(* Logix 5000 AddOnInstructionDefinition export B256_CtoS; software revision 30.00 *)

ADD_ON_INSTRUCTION D_SHR   (* revision 1.0, vendor Ken Fischer, NSWCPD, C512 *)
// DINT bit shift right of the 32-bit argument Inp_A by Inp_B bits with paddding by zeros on the right
// Revision note:
// Rev1.0: TBD - Initial Release
VAR_IN_OUT
   Inp_A : DINT; {required}   // 64-bit Integer to be right circular rotated
END_VAR
VAR_INPUT
   Inp_B : INT; {required}   // Number of bits to shift
END_VAR
VAR_IN_OUT
   Out : DINT; {required}   // Result
END_VAR
VAR
   BSR_Cntrl : CONTROL := (LEN := 32);
   ONS : BOOL;
   Source_Bit : BOOL;
   Wrk_InpA : DINT[2];
END_VAR

ROUTINE Logic   (* ladder *)
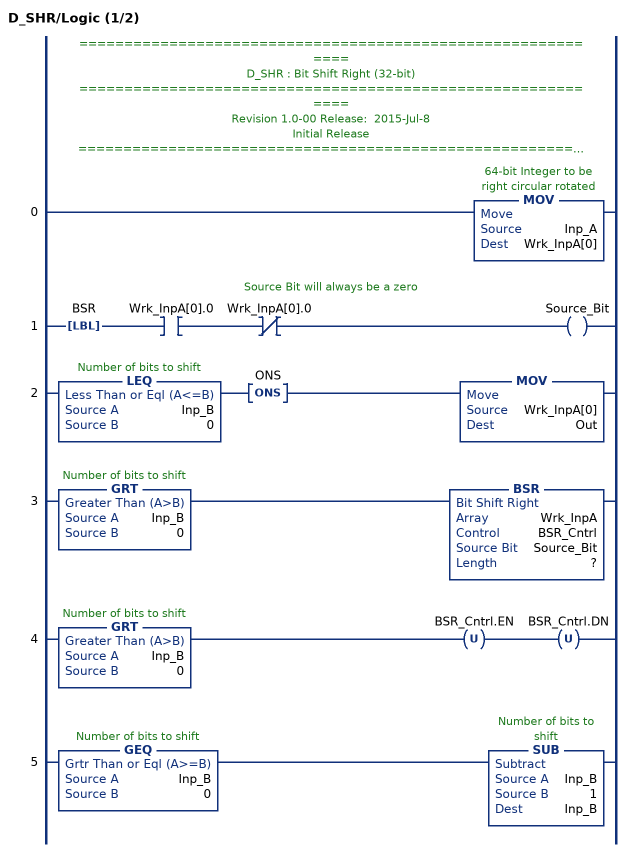
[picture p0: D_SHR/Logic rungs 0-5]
   // ============================================================
   // D_SHR : Bit Shift Right (32-bit)
   // ============================================================
   // Revision 1.0-00 Release:  2015-Jul-8
   // Initial Release
   // ============================================================
   // Performs a right bit shift of the 32-bit argument Inp_A by the
   // number of bits defined in the 16-bit argument Inp_B, with padding by zeros.
   0: MOV(Inp_A,Wrk_InpA[0]);
   // Source Bit will always be a zero
   1: LBL(BSR)XIC(Wrk_InpA[0].0)XIO(Wrk_InpA[0].0)OTE(Source_Bit);
   2: LEQ(Inp_B,0)ONS(ONS)MOV(Wrk_InpA[0],Out);
   3: GRT(Inp_B,0)BSR(Wrk_InpA,BSR_Cntrl,Source_Bit,?);
   4: GRT(Inp_B,0)OTU(BSR_Cntrl.EN)OTU(BSR_Cntrl.DN);
   5: GEQ(Inp_B,0)SUB(Inp_B,1,Inp_B);
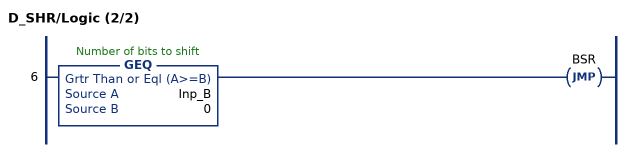
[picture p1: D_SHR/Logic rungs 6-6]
   6: GEQ(Inp_B,0)JMP(BSR);
END_ROUTINE
END_ADD_ON_INSTRUCTION

ADD_ON_INSTRUCTION B256_CtoS   (* revision 1.0 20170916, vendor Kenneth A. Fischer *)
// Convert 256-bit value using 22 12-bit pieces into 64 hex big endian string characters
// Revision note:
// Rev1.0: 20170916 - Initial Release
VAR_IN_OUT
   Inp_C : DINT[22]; {required}
   Out_S : STRING; {required}
END_VAR
VAR
   byte : DINT[3];
   i : INT;
   j : INT;
   k : DINT;
   D_SHR : D_SHR;
END_VAR

ROUTINE Logic   (* ladder *)
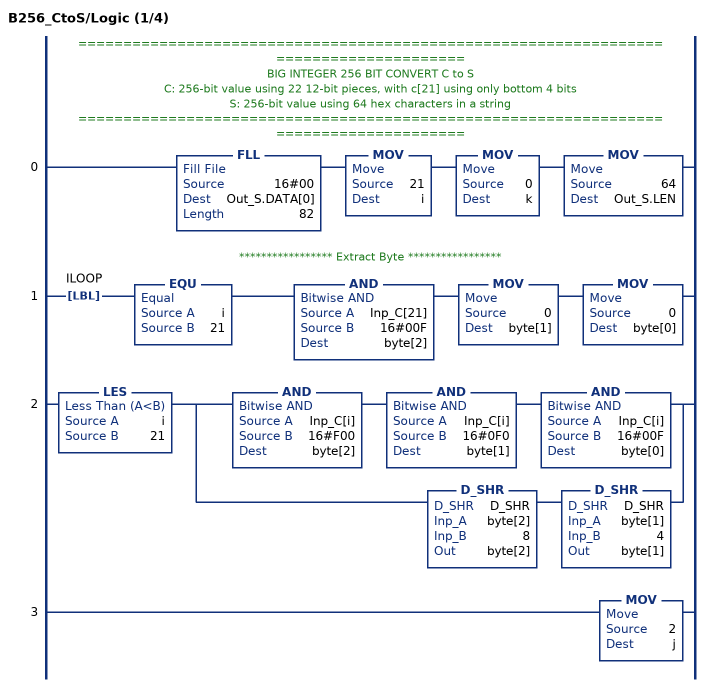
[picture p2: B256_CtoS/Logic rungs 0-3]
   // ======================================================================================
   // BIG INTEGER 256 BIT CONVERT C to S
   // C: 256-bit value using 22 12-bit pieces, with c[21] using only bottom 4 bits
   // S: 256-bit value using 64 hex characters in a string
   // ======================================================================================
   0: FLL(16#00,Out_S.DATA[0],82)MOV(21,i)MOV(0,k)MOV(64,Out_S.LEN);
   // ***************** Extract Byte *****************
   1: LBL(ILOOP)EQU(i,21)AND(Inp_C[21],16#00F,byte[2])MOV(0,byte[1])MOV(0,byte[0]);
   2: LES(i,21)[AND(Inp_C[i],16#F00,byte[2]) AND(Inp_C[i],16#0F0,byte[1]) AND(Inp_C[i],16#00F,byte[0]) ,D_SHR(D_SHR,byte[2],8,byte[2]) D_SHR(D_SHR,byte[1],4,byte[1]) ];
   3: MOV(2,j);
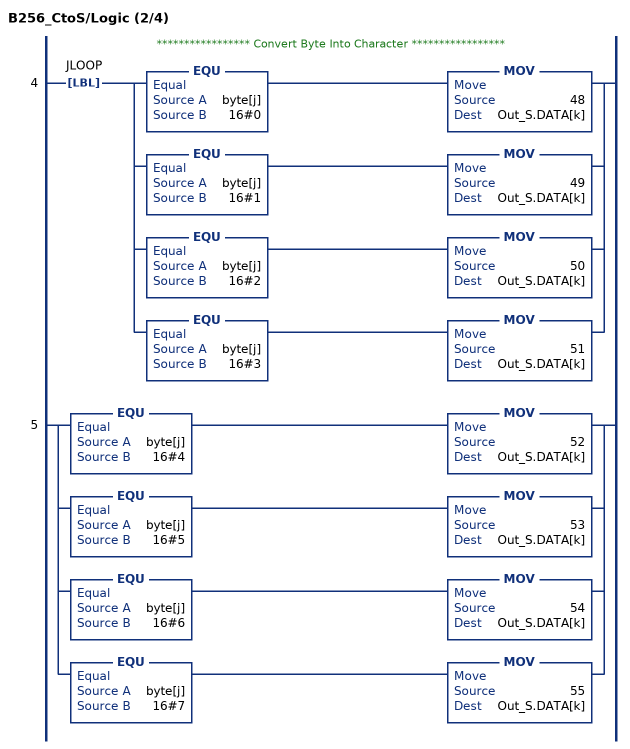
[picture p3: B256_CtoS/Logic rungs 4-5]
   // ***************** Convert Byte Into Character *****************
   4: LBL(JLOOP)[EQU(byte[j],16#0) MOV(48,Out_S.DATA[k]) ,EQU(byte[j],16#1) MOV(49,Out_S.DATA[k]) ,EQU(byte[j],16#2) MOV(50,Out_S.DATA[k]) ,EQU(byte[j],16#3) MOV(51,Out_S.DATA[k]) ];
   5: [EQU(byte[j],16#4) MOV(52,Out_S.DATA[k]) ,EQU(byte[j],16#5) MOV(53,Out_S.DATA[k]) ,EQU(byte[j],16#6) MOV(54,Out_S.DATA[k]) ,EQU(byte[j],16#7) MOV(55,Out_S.DATA[k]) ];
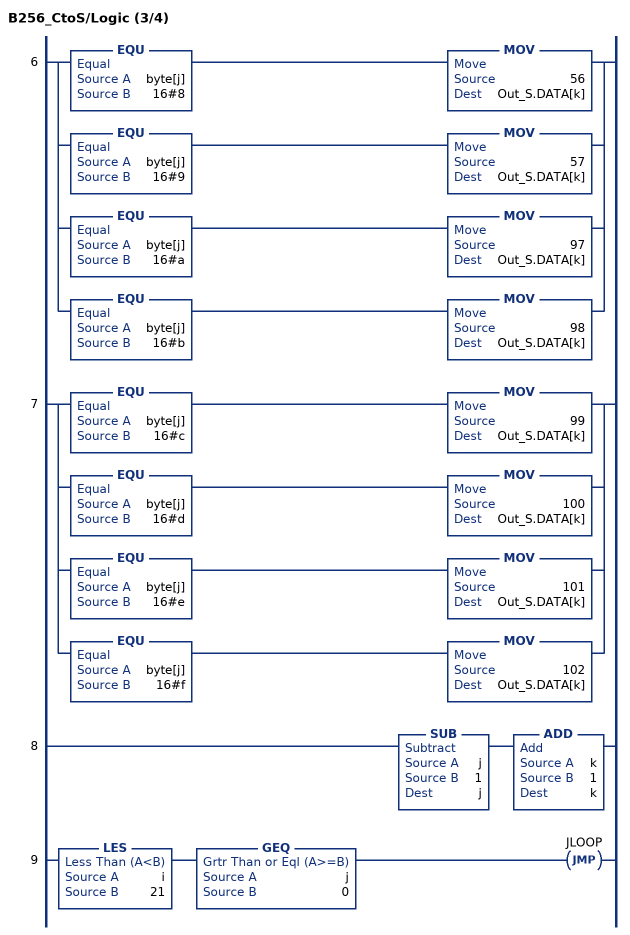
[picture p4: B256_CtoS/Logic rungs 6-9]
   6: [EQU(byte[j],16#8) MOV(56,Out_S.DATA[k]) ,EQU(byte[j],16#9) MOV(57,Out_S.DATA[k]) ,EQU(byte[j],16#a) MOV(97,Out_S.DATA[k]) ,EQU(byte[j],16#b) MOV(98,Out_S.DATA[k]) ];
   7: [EQU(byte[j],16#c) MOV(99,Out_S.DATA[k]) ,EQU(byte[j],16#d) MOV(100,Out_S.DATA[k]) ,EQU(byte[j],16#e) MOV(101,Out_S.DATA[k]) ,EQU(byte[j],16#f) MOV(102,Out_S.DATA[k]) ];
   8: SUB(j,1,j)ADD(k,1,k);
   9: LES(i,21)GEQ(j,0)JMP(JLOOP);
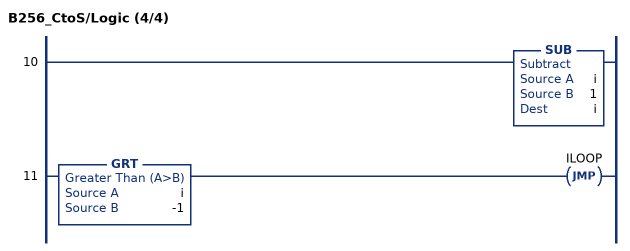
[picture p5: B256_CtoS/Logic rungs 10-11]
   10: SUB(i,1,i);
   11: GRT(i,-1)JMP(ILOOP);
END_ROUTINE
END_ADD_ON_INSTRUCTION
